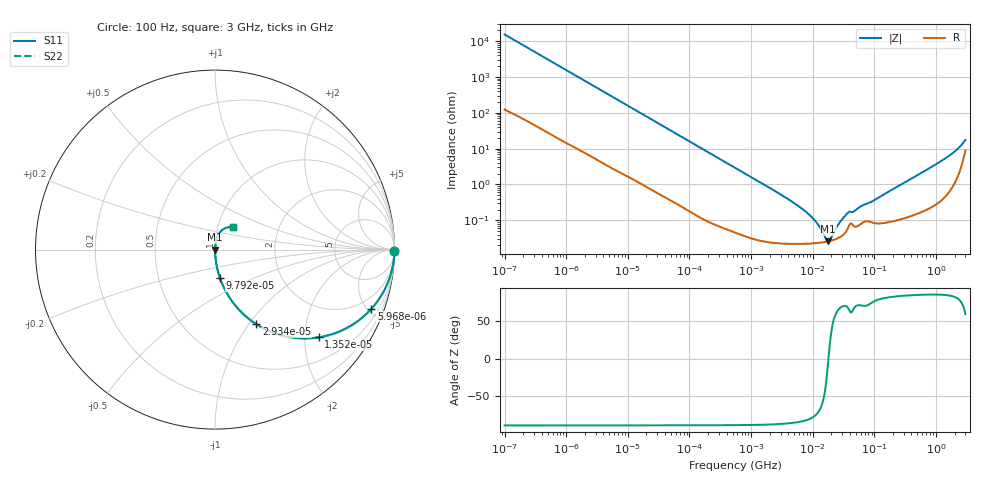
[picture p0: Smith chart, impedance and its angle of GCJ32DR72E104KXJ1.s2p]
!Murata Part Number: GCJ32DR72E104KXJ1
!These Parameters are Measured in Series Mode Connection
!Data Generated on Mar 13, 2026
!  o--ll--o
!Port1  Port2
!  o------o
!Operation Temp=25[degC], DC Bias Voltage=0[V]
!Freq. Start=100[Hz] Stop=3[GHz] 401[Steps]
# Hz S RI R 50
!Freq.(Hz) S11(Real) S11(Imag) S21(Real) S21(Imag) S12(Real) S12(Imag) S22(Real) S22(Imag)
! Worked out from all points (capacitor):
!   401 points, 100 Hz to 3 GHz, reference 50 ohm
!   read as one part in series: C = 103 nF near 109 Hz
!   lowest |Z| = 26 mohm at 17.89 MHz (marker M1)
!   series resonance near 17.98 MHz, so ESL is about 760 pH
!   S11 on the Smith chart (normalised r, x): 100 Hz: open; 5.968 kHz: 1.05, -5.28; 13.52 kHz: 1.03, -2.34; 29.34 kHz: 1.01, -1.08; 97.92 kHz: 1.00, -0.33; 3 GHz: 1.18, +0.30
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100  0.9999 -0.00651  9.46e-05 0.00651  9.46e-05 0.00651  0.9999 -0.00651
584  0.9982 -0.0375  0.00175 0.0375  0.00175 0.0375  0.9982 -0.0375
1788  0.986 -0.1127  0.014 0.1127  0.014 0.1127  0.986 -0.1127
5968  0.8719 -0.3293  0.1281 0.3293  0.1281 0.3293  0.8719 -0.3293
13520  0.5774 -0.4887  0.4226 0.4887  0.4226 0.4887  0.5774 -0.4887
29339  0.2298 -0.4153  0.7702 0.4153  0.7702 0.4153  0.2298 -0.4153
31977  0.2013 -0.3956  0.7987 0.3956  0.7987 0.3956  0.2013 -0.3956
53598  0.0842 -0.2722  0.9158 0.2722  0.9158 0.2722  0.0842 -0.2722
97915  0.0278 -0.1591  0.9722 0.1591  0.9722 0.1591  0.0278 -0.1591
547723  0.00133 -0.0295  0.9987 0.0295  0.9987 0.0295  0.00133 -0.0295
4323298  0.000233 -0.00355  0.9998 0.00355  0.9998 0.00355  0.000233 -0.00355
9794414  0.000227 -0.00117  0.9998 0.00117  0.9998 0.00117  0.000227 -0.00117
1.268047e7  0.000236 -0.000648  0.9998 0.000648  0.9998 0.000648  0.000236 -0.000648
1.641694e7  0.000251 -0.000166  0.9997 0.000166  0.9997 0.000166  0.000251 -0.000166
1.789277e7  0.000259 -9.2e-06  0.9997 9.2e-06  0.9997 9.2e-06  0.000259 -9.2e-06
1.950129e7  0.000269 0.000148  0.9997 -0.000148  0.9997 -0.000148  0.000269 0.000148
2.751729e7  0.000338 0.000813  0.9997 -0.000813  0.9997 -0.000813  0.000338 0.000813
3.71925e7  0.000607 0.00151  0.9994 -0.00151  0.9994 -0.00151  0.000607 0.00151
4.815176e7  0.000666 0.00172  0.9993 -0.00172  0.9993 -0.00172  0.000666 0.00172
1.751444e8  0.000932 0.0064  0.9991 -0.0064  0.9991 -0.0064  0.000932 0.0064
1.324213e9  0.00645 0.0489  0.9936 -0.0489  0.9936 -0.0489  0.00645 0.0489
3e9  0.0984 0.1242  0.9016 -0.1242  0.9016 -0.1242  0.0984 0.1242
